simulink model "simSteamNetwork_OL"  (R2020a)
settings: Solver=ode15s  StartTime=0.0  StopTime=tsim  RelTol=1e-8
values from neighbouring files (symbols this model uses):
  d0 = [Fh, Tcin, Thin]    [Main.m]    (also in Main_OL.m; runTestCalcBlk.m; runTransf.m = [Fh, Tcin, Thin,U0]; runTransfOL.m)
  dd = 0    [Main.m]
  du = [0.; 0.05]    [Main.m]
  nd = size(d0,2)    [Main.m]    (also in Main_OL.m; runTestCalcBlk.m; runTransf.m; runTransfOL.m)
  np = size(p,2)    [Main.m]    (also in runH2Psim.m = length(param); Main_OL.m; runTestCalcBlk.m; runTransf.m)
  nu = 1    [Main.m]    (also in runH2Psim.m = length(u0); Main_OL.m; runTestCalcBlk.m; runTransf.m)
  nx = size(x0,1)    [Main.m]    (also in H2P_Turbine_driven.m = param(end); runTD.m = length(x0); H2P_Boiler_driven.m = param(end); runBD.m = length(x0))
  param = [R;gamma;VH;VL;phi;CvH;CvHC;CvTB;CvLC1;CvLC2;AH;AL]    [Main.m]    (also in runTD.m = [Tref;TrefB;dHvap;cpg;cpW;cpSt;R;Mwt;     T0;TG0;ME;pC;     ; runBD.m = [Tref;TrefB;dHvap;cpg;cpW;cpSt;R;Mwt;          T0;TG0;ME;pC;; runFP.m = [Tref;TrefB;dHvap;cpg;cpW;cpSt;R;Mwt;          T0;TG0;ME;pC;; runFPV2.m = [Tref;TrefB;dHvap;cpg;cpW;cpSt;R;Mwt;          T0;TG0;ME;pC;)
  td = 0    [Main.m]
  tu = 10    [Main.m]
  u0 = [z0;z0]    [Main.m]    (also in runH2Psim.m = [mG0;zV0;mP0;mB0;mA0]; calcblock.m = p(2); testfun.m = 5; u_function.m = 5)
  x0 = [Tcend(1:N)'; Thend(1:N)']    [Main.m]    (also in runTD.m = [TE0;TD0;TSh0;MD0; MSh0;w0;TA0;0;0;0;0;0;0;0;0;0]; runBD.m = [TE0;TD0;TSh0;MD0; MSh0;w0;TA0;0;0;0;0;0;0;0;0;0]; runFP.m = [TE0;TD0;TSh0;MD0; MSh0;w0;TA0;0;0;0;0;0;0;0]; runFPV2.m = [TE0;TD0;TSh0;MD0; MSh0;w0;TA0;0;0;0;0;0;0;0])
undefined symbols (not defined in the file or in its folder): SteamNetwork

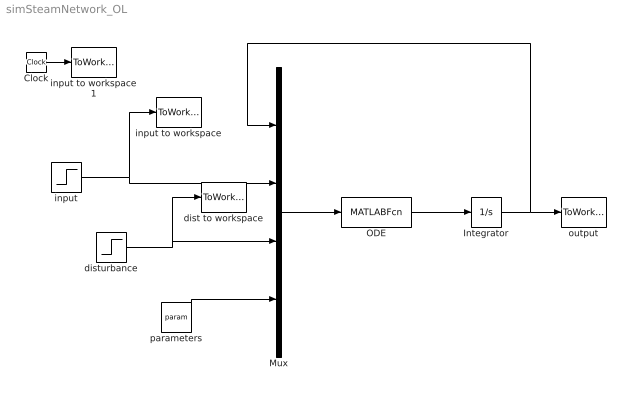
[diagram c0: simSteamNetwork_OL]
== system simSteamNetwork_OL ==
  Clock : Clock
  Integrator : Integrator  InitialCondition=x0
  Mux : Mux
  ODE : MATLABFcn  MATLABFcn=SteamNetwork(u(1:nx),(u(nx+1:nx+nu)),u(nx+nu+1:nx+nu+nd),u(nx+nu+nd+1:nx+nu+nd+np))
  dist to workspace : ToWorkspace  VariableName=d  SampleTime=-1
  disturbance : Step  Time=td  Before=d0  After=d0+dd  SampleTime=0
  input : Step  Time=tu  Before=u0  After=u0+du  SampleTime=0
  input to workspace : ToWorkspace  VariableName=u  SampleTime=-1
  input to workspace1 : ToWorkspace  VariableName=time  SampleTime=-1
  output : ToWorkspace  VariableName=y  SampleTime=-1
  parameters : Constant  Value=param
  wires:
  ODE/1 -> Integrator/1
  Integrator/1 -> Mux/1, output/1
  Mux/1 -> ODE/1
  input/1 -> input to workspace/1, Mux/2
  disturbance/1 -> dist to workspace/1, Mux/3
  parameters/1 -> Mux/4
  Clock/1 -> input to workspace1/1
